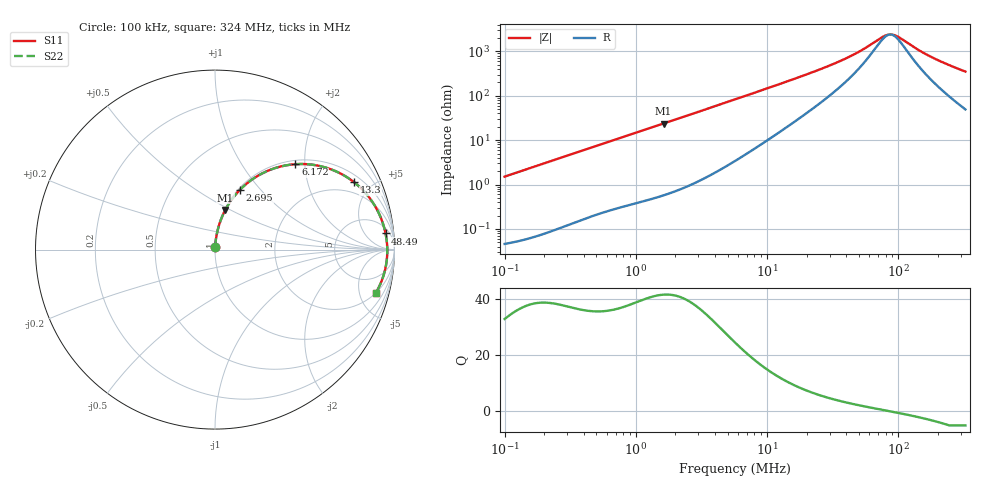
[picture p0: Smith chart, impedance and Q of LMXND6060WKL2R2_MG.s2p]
! LMXND6060WKL2R2_MG  S-PARAMETER MODEL  ( General Type )
! Model Generated by TAIYO YUDEN Corporation (https://www.yuden.co.jp/en/)
! Version 1.0
! TAIYO YUDEN Control No. 191025NI43SB-FBB
! Copyright(c) 2019 TAIYO YUDEN CO.,LTD. All Rights Reserved.
! Product Description (link to TY-COMPAS)
! https://ds.yuden.co.jp/TYCOMPAS/or/detail?pn=LMXND6060WKL2R2NMG&u=M
! Products Name : Inductors
! Characteristics :
!  Inductance : 2.2 uH , SRF(min) : 73 MHz , DC Resistance(max) : 0.0408 Ohm
!  Rated Current : Saturation :3200 mA , Temp Rise : 2900 mA (40 degC)
!  Case Size : 6.0 x 6.0 / 0.236 x 0.236 [mm/inch] , Thickness : 2 / 0.079 [mm/inch]
!  (Conditions: Temperature = 25 degC , DC Bias Current/Voltage = 0A / 0V)
! External Node Assignments :
!  1  o---GGG---o  2
! GND o---------o GND
! Frequency Range : 0.1MHz  -  324.04089MHz  [ 402 STEP ]
# MHz S RI R 50
! Freq[MHz].  S11 Real  S11 Imag  S21 Real  S21 Imag  S12 Real  S12 Imag  S22 Real  S22 Imag
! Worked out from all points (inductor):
!   401 points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, 100 kHz to 324 MHz, reference 50 ohm
!   read as one part in series: L = 2.39 uH near 104.1 kHz
!   highest Q = 41.4 at 1.626 MHz (marker M1), where L = 2.31 uH
!   self-resonance near 86.74 MHz
!   S11 on the Smith chart (normalised r, x): 100 kHz: 1.00, +0.03; 2.695 MHz: 1.02, +0.78; 6.172 MHz: 1.08, +1.79; 13.3 MHz: 1.35, +3.91; 48.49 MHz: 8, +17; 324 MHz: 1.98, -6.92
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0.1  0.000686 0.015  0.9993 -0.015  0.9993 -0.015  0.000686 0.015
0.38728  0.00489 0.0572  0.9951 -0.0572  0.9951 -0.0572  0.00489 0.0572
0.80164  0.0167 0.1152  0.9833 -0.1152  0.9833 -0.1152  0.0167 0.1152
1.499861  0.05 0.2061  0.95 -0.2061  0.95 -0.2061  0.05 0.2061
1.626136  0.0577 0.2214  0.9423 -0.2214  0.9423 -0.2214  0.0577 0.2214
2.695066  0.139 0.3332  0.861 -0.3332  0.861 -0.3332  0.139 0.3332
3.877452  0.2472 0.4161  0.7528 -0.4161  0.7528 -0.4161  0.2472 0.4161
5.692459  0.4099 0.4718  0.5901 -0.4718  0.5901 -0.4718  0.4099 0.4718
6.171716  0.4483 0.4759  0.5517 -0.4759  0.5517 -0.4759  0.4483 0.4759
8.701746  0.6109 0.4589  0.3891 -0.4589  0.3891 -0.4589  0.6109 0.4589
13.30188  0.7742 0.376  0.2258 -0.376  0.2258 -0.376  0.7742 0.376
22.04577  0.8874 0.2496  0.1126 -0.2496  0.1126 -0.2496  0.8874 0.2496
34.38811  0.9334 0.1522  0.0666 -0.1522  0.0666 -0.1522  0.9334 0.1522
48.48516  0.9503 0.09  0.0497 -0.09  0.0497 -0.09  0.9503 0.09
75.62961  0.9593 0.0205  0.0407 -0.0205  0.0407 -0.0205  0.9593 0.0205
85.37896  0.9599 0.00236  0.0401 -0.00236  0.0401 -0.00236  0.9599 0.00236
90.71526  0.96 -0.00669  0.04 0.00669  0.04 0.00669  0.96 -0.00669
98.35271  0.9598 -0.0188  0.0402 0.0188  0.0402 0.0188  0.9598 -0.0188
141.5022  0.9547 -0.076  0.0453 0.076  0.0453 0.076  0.9547 -0.076
187.7735  0.9443 -0.1259  0.0557 0.1259  0.0557 0.1259  0.9443 -0.1259
249.1755  0.925 -0.1832  0.075 0.1832  0.075 0.1832  0.925 -0.1832
324.0409  0.895 -0.2437  0.105 0.2437  0.105 0.2437  0.895 -0.2437
